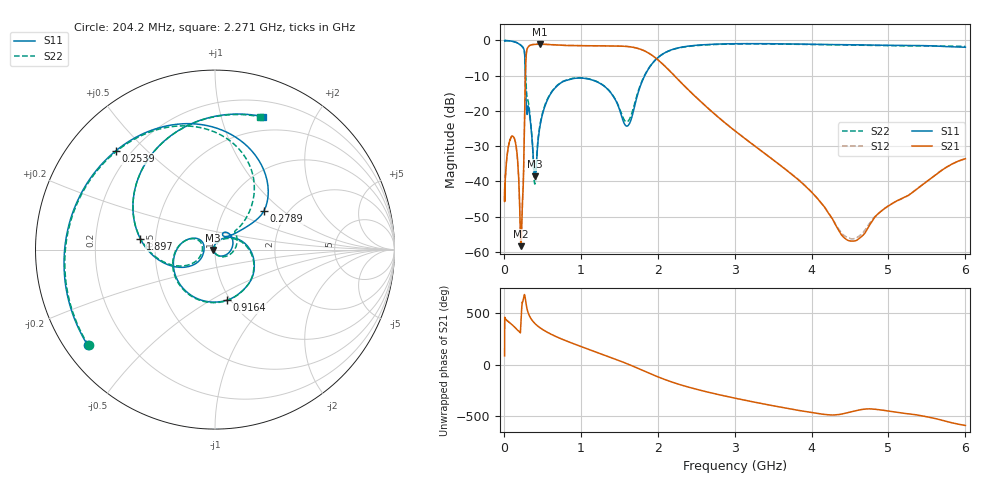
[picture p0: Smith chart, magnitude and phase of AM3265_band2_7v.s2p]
!Agilent Technologies,E8364B,MY43040894,A.07.50.67
!Agilent E8364B: A.07.50.67
!Date: Friday, May 09, 2025 07:25:47
!Correction: S11(Full 2 Port(1,2))
!S21(Full 2 Port(1,2))
!S12(Full 2 Port(1,2))
!S22(Full 2 Port(1,2))
!S2P File: Measurements: S11, S21, S12, S22:Log Frequency Sweep
# Hz S  dB  R 50
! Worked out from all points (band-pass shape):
!   3201 points, 10 MHz to 6 GHz, reference 50 ohm
!   highest |S21| = -1.07 dB at 464.4 MHz (marker M1); lowest = -58.4 dB at 222.1 MHz (marker M2)
!   |S21| within 3 dB of the highest: 291.2 MHz to 1.918 GHz (1.626 GHz wide, 147 % of centre)
!   lowest |S11| = -38.5 dB at 403.8 MHz (marker M3), VSWR 1.02, Z = 48.9 - j0.214 ohm
!   |S11| at or under -10 dB: 279.6 MHz to 1.831 GHz (1.552 GHz wide, 147 % of centre)
!   |S22| runs from -40.7 to 0.0 dB; largest |S21 - S12| = 0.014
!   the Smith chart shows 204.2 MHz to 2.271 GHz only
!   S11 on the Smith chart (normalised r, x): 204.2 MHz: 0.07, -0.33; 253.9 MHz: 0.14, +0.40; 278.9 MHz: 1.53, +0.74; 916.4 MHz: 0.96, -0.59; 1.897 GHz: 0.41, +0.06; 2.271 GHz: 0.35, +1.36
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1e7  -0.03 -5.4  -45.45 86.6  -41.69 58.8  -0.07 -5.6
2.908064e7  -0.04 -15.9  -35.90 76.2  -35.53 75.4  -0.05 -15.9
8.439949e7  -0.12 -47.4  -28.04 41.8  -28.03 42.3  -0.16 -47.7
2.042076e8  -1.04 -143.2  -45.71 -41.0  -45.51 -42.2  -1.07 -142.9
2.220932e8  -1.35 -166.2  -58.38 46.6  -58.02 96.2  -1.38 -165.2
2.44949e8  -1.87 155.5  -44.68 -114.0  -44.43 -114.2  -1.88 158.1
2.539234e8  -2.16 135.2  -39.67 -78.7  -39.70 -78.7  -2.14 139.3
2.789374e8  -9.21 38.3  -10.67 -77.2  -10.64 -77.2  -7.19 60.2
3.088756e8  -19.13 61.0  -2.09 160.0  -2.05 160.0  -16.73 38.7
4.037557e8  -38.54 -169.3  -1.11 39.6  -1.07 39.6  -40.73 176.4
4.643984e8  -25.07 66.6  -1.07 1.2  -1.04 1.3  -24.62 59.2
7.123273e8  -12.52 -22.1  -1.31 -98.4  -1.27 -98.4  -12.40 -25.6
9.163667e8  -10.76 -76.9  -1.47 -159.4  -1.43 -159.4  -10.67 -79.7
1.337069e9  -13.57 178.2  -1.54 85.6  -1.51 85.6  -13.50 178.0
1.897073e9  -7.51 171.6  -3.78 -84.0  -3.76 -84.0  -7.42 170.5
2.067357e9  -3.82 121.7  -6.74 -136.0  -6.72 -136.0  -3.83 122.0
2.271013e9  -2.07 70.2  -11.22 171.4  -11.19 171.5  -2.14 71.1
3.202913e9  -0.90 -91.4  -28.99 6.1  -28.98 6.1  -0.97 -91.5
3.818953e9  -1.02 -178.2  -39.36 -80.4  -39.28 -80.7  -1.08 -179.7
4.499191e9  -1.22 90.8  -56.87 -100.0  -56.20 -100.8  -1.30 89.3
5.195685e9  -1.41 -0.2  -44.61 -109.8  -44.68 -110.5  -1.52 -0.1
6e9  -1.92 -97.0  -33.55 132.1  -33.60 131.7  -1.67 -96.5
